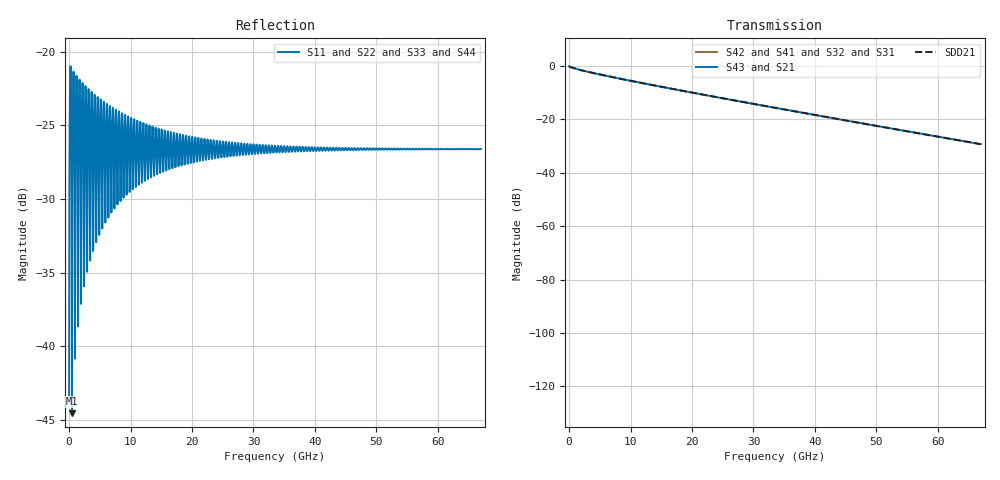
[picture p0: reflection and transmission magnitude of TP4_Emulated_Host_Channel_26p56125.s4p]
! Created Tue Oct  9 18:05:27 2018
# hz S ma R 50
! 4 Port Network Data from SP1.SP block
! freq  magS11  angS11  magS12  angS12  magS13  angS13  magS14  angS14
!  magS21  angS21  magS22  angS22  magS23  angS23  magS24  angS24
!  magS31  angS31  magS32  angS32  magS33  angS33  magS34  angS34
!  magS41  angS41  magS42  angS42  magS43  angS43  magS44  angS44
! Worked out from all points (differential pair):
!   6700 points, 10 MHz to 67 GHz, reference 50 ohm
!   strongest paths, dB at 10 MHz, 16.76 GHz, 33.51 GHz, 50.26 GHz, 67 GHz:
!     S43: -0.1, -8.5, -15.7, -22.5, -29.3
!     S21: -0.1, -8.5, -15.7, -22.5, -29.3
!     S42: -180.0, -180.0, -180.0, -180.0, -180.0
!     S41: -180.0, -180.0, -180.0, -180.0, -180.0
!     S32: -180.0, -180.0, -180.0, -180.0, -180.0
!     S31: -180.0, -180.0, -180.0, -180.0, -180.0
!   taken as a pair (ports 3,1 in; 4,2 out), SDD21 dB: -0.1, -8.5, -15.7, -22.5, -29.3
!   lowest |S11| = -44.6 dB at 480 MHz (marker M1), VSWR 1.01, Z = 50.6 - j0.0571 ohm
!   |S11| at or under -10 dB: start of sweep to end of sweep
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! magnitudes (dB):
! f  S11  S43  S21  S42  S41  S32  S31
! 10 MHz  -43.4  -0.1  -0.1  -180.0  -180.0  -180.0  -180.0
! 480 MHz  -44.6  -0.6  -0.6  -180.0  -180.0  -180.0  -180.0
! 730 MHz  -21.3  -0.8  -0.8  -180.0  -180.0  -180.0  -180.0
! 960 MHz  -39.8  -0.9  -0.9  -180.0  -180.0  -180.0  -180.0
! 1.22 GHz  -21.6  -1.1  -1.1  -180.0  -180.0  -180.0  -180.0
! 1.45 GHz  -38.0  -1.2  -1.2  -180.0  -180.0  -180.0  -180.0
! 67 GHz  -26.6  -29.3  -29.3  -180.0  -180.0  -180.0  -180.0
